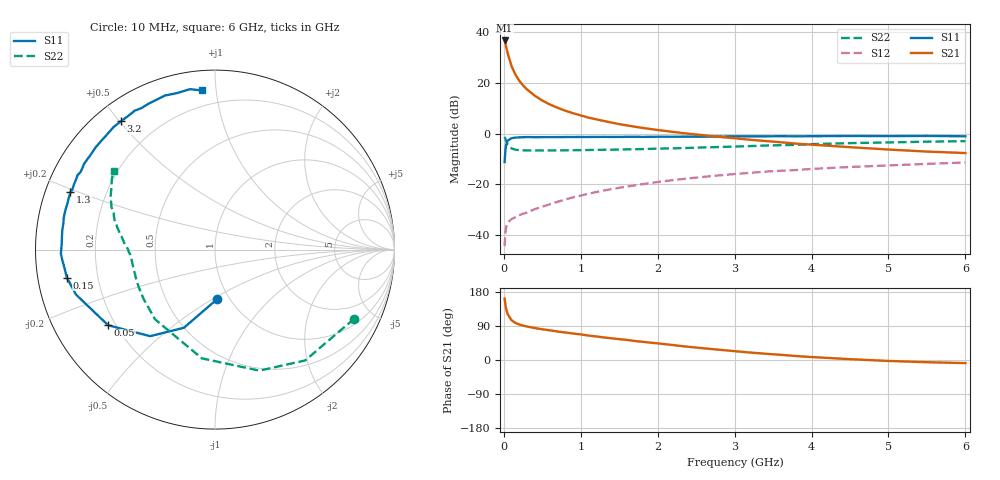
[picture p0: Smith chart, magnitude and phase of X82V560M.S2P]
! SIEMENS Small Signal Semiconductors
! BFP136W
! Si NPN RF Bipolar Junction Transistor in SOT343
! VCE = 2.5 V  IC = 60 mA
! Common Emitter S-Parameters:  September  1994
# GHz  S  MA  R  50
!  f  S11  S21  S12  S22
! GHz  MAG  ANG  MAG  ANG  MAG  ANG  MAG  ANG
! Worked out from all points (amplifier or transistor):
!   40 points, 10 MHz to 6 GHz, reference 50 ohm
!   highest |S21| = 36.9 dB at 10 MHz (marker M1)
!   |S21| within 3 dB of that: start of sweep to 34.27 MHz
!   unconditionally stable (mu >= 1): 580.1 MHz to 2.88 GHz
!   at 200 MHz: K = 0.59, MSG = 26.6 dB, |S12| = -32.3 dB
!   at 1.5 GHz: K = 1.11, MAG = 10.6 dB, |S12| = -21.4 dB
!   at 6 GHz: K = 0.97, MSG = 1.9 dB, |S12| = -11.4 dB
!   S11 on the Smith chart (normalised r, x): 10 MHz: 0.88, -0.52; 50 MHz: 0.17, -0.31; 150 MHz: 0.09, -0.09; 1.3 GHz: 0.07, +0.19; 3.2 GHz: 0.08, +0.51; 6 GHz: 0.11, +0.92
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0.01  0.2758 -87.4  69.62 162.1  0.006 70.8  0.8661 -26.4
0.02  0.4687 -111.7  61.22 146.6  0.011 58.8  0.7959 -50.9
0.03  0.603 -126.9  52.7 135.2  0.0141 50.5  0.7181 -69.9
0.05  0.7295 -144.7  38.52 120.6  0.0175 38.7  0.6102 -96.9
0.1  0.8142 -162.1  21.7 105.0  0.0206 32.8  0.5123 -130.7
0.15  0.8401 -169.3  14.82 98.0  0.0224 34.7  0.4833 -145.6
0.2  0.8453 -173.2  11.15 93.7  0.0244 36.7  0.4736 -153.8
0.25  0.8534 -176.4  8.997 90.7  0.0263 38.9  0.4698 -159.0
0.3  0.8589 -178.4  7.529 88.4  0.0277 41.4  0.4664 -162.6
0.4  0.8546 177.7  5.671 84.4  0.0323 46.3  0.4661 -167.2
0.5  0.856 174.9  4.521 81.0  0.0361 50.1  0.4665 -170.2
0.6  0.8577 172.7  3.771 78.3  0.0405 52.1  0.4674 -172.2
0.7  0.8573 170.1  3.25 75.1  0.0453 55.0  0.4689 -173.5
0.9  0.8616 166.7  2.541 69.9  0.0553 57.1  0.4718 -176.0
1.1  0.8615 162.3  2.082 64.4  0.065 58.5  0.4769 -177.6
1.3  0.8663 158.4  1.789 59.5  0.0755 58.9  0.4821 -179.2
1.7  0.8706 151.5  1.379 50.2  0.0954 57.8  0.4944 177.8
2.2  0.871 143.2  1.085 39.4  0.121 54.8  0.5141 174.2
3.2  0.8864 126.2  0.76 19.7  0.1688 46.1  0.5692 165.3
4.5  0.9024 108.0  0.542 2.2  0.2201 34.0  0.6521 153.1
5.5  0.9047 98.9  0.444 -5.8  0.2534 26.0  0.6966 145.6
6  0.8895 94.6  0.415 -8.2  0.2701 21.6  0.7132 142.4
